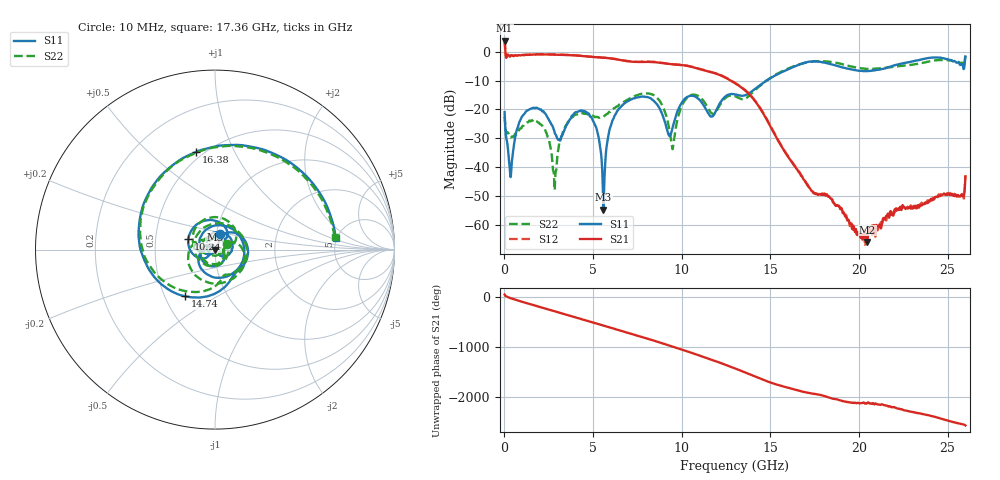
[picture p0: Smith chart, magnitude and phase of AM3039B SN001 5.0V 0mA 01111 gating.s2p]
!Agilent Technologies,E8364B,MY43040894,A.07.50.67
!Agilent E8364B: A.07.50.67
!Date: Tuesday, June 28, 2016 08:06:53
!Correction: S11(Full 2 Port(1,2))
!S21(Full 2 Port(1,2))
!S12(Full 2 Port(1,2))
!S22(Full 2 Port(1,2))
!S2P File: Measurements: S11, S21, S12, S22:
# Hz S  dB  R 50
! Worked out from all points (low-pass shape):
!   1601 points, 10 MHz to 26 GHz, reference 50 ohm
!   highest |S21| = 3.74 dB at 10 MHz (marker M1); lowest = -65.7 dB at 20.48 GHz (marker M2)
!   |S21| within 3 dB of the highest: start of sweep to 44.06 MHz
!   lowest |S11| = -54.6 dB at 5.582 GHz (marker M3), VSWR 1.00, Z = 49.8 + j0.0303 ohm
!   |S11| at or under -10 dB: start of sweep to 14.79 GHz
!   |S22| runs from -47.8 to -1.1 dB; largest |S21 - S12| = 0.028
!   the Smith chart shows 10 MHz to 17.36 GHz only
!   S11 on the Smith chart (normalised r, x): 10 MHz: 1.04, +0.18; 10.24 GHz: 0.74, +0.09; 14.74 GHz: 0.63, -0.36; 16.38 GHz: 0.46, +0.72; 17.36 GHz: 4.90, +1.12
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1e7  -20.91 72.2  3.74 40.9  3.82 41.8  -22.36 24.3
7.24725e8  -26.61 148.3  -1.45 -73.9  -1.40 -73.7  -28.16 -160.1
1.683106e9  -19.51 48.0  -1.03 -173.6  -1.00 -173.5  -23.67 49.3
2.722706e9  -25.93 -46.8  -1.05 80.5  -0.99 80.6  -39.77 -65.5
3.51865e9  -25.19 -30.0  -1.22 -0.7  -1.16 -0.5  -25.07 -23.1
4.347081e9  -20.51 -114.7  -1.52 -86.3  -1.49 -86.2  -21.35 -139.5
5.581606e9  -54.58 170.6  -2.14 145.8  -2.08 145.9  -22.46 -20.1
6.946081e9  -17.20 80.0  -3.35 2.8  -3.29 3.1  -16.63 84.8
8.684162e9  -18.93 -144.5  -3.79 178.2  -3.70 178.7  -16.46 -170.4
1.024356e10  -15.96 159.0  -4.86 1.7  -4.78 2.1  -16.35 142.3
1.165677e10  -22.42 50.6  -7.13 -168.3  -7.04 -167.8  -21.09 16.0
1.3005e10  -14.76 -23.6  -10.94 14.6  -10.82 15.2  -15.42 -48.6
1.474308e10  -10.19 -122.9  -22.91 128.0  -22.69 128.3  -10.22 -135.6
1.63837e10  -5.11 100.7  -39.66 -47.2  -39.47 -46.7  -4.94 92.4
1.734208e10  -3.41 6.9  -48.14 -124.8  -47.98 -125.0  -3.49 7.4
1.735832e10  -3.41 5.3  -48.22 -125.9  -48.14 -126.0  -3.47 5.9
1.84629e10  -4.47 -102.1  -50.98 139.0  -50.90 139.8  -3.63 -93.1
2.047712e10  -6.76 101.6  -65.68 49.8  -62.89 55.5  -5.96 111.0
2.167916e10  -5.36 19.6  -57.00 -22.2  -57.52 -14.6  -5.46 25.5
2.317359e10  -3.15 -92.9  -53.61 -140.2  -53.75 -146.6  -4.37 -83.3
2.427816e10  -2.07 177.4  -50.36 133.9  -50.27 132.4  -3.10 -167.5
2.6e10  -1.81 -18.5  -43.21 -37.6  -42.63 -35.5  -1.11 12.1
